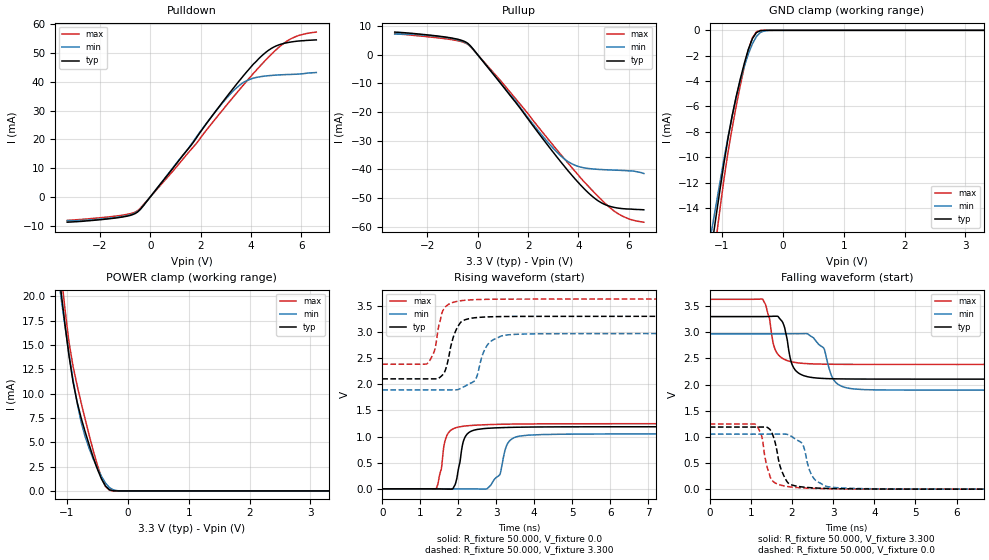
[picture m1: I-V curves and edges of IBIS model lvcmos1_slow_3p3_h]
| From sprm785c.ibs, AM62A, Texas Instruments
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|   slow_3p3_h
[Model]   lvcmos1_slow_3p3_h
Model_type I/O
Polarity   Non-Inverting
Enable   Active-High
Vinl = 0
Vinh = 0.8
Vmeas = 1.65
Vref = 3.3
Cref = 2pF
Rref = 100000
|   typ   min   max
C_comp   3.477pF   3.396pF   3.491pF
[Voltage Range]   3.3   2.97   3.63
[Temperature Range]   27   150   -40
[Pullup Reference]   3.3   2.97   3.63
[Pulldown Reference]   0   0   0
[Power Clamp Reference]   3.3   2.97   3.63
[GND Clamp Reference]   0   0   0
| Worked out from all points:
|   slope of the pulldown table from 0 to 0.495 V, typ, clamps not added: 90.3 ohm
|   slope of the pullup table from 0 to 0.495 V, typ, clamps not added: 91.7 ohm
|   GND clamp passes 1 mA (typ) near -0.53 V on its own axis
|   POWER clamp passes 1 mA (typ) near -0.41 V on its own axis
|   rising waveform, R_fixture 50.000, V_fixture 0.0: 20-80 % time 183ps typ, 292ps min, 182ps max; typ from 0 V to 1.19 V
|   rising waveform, R_fixture 50.000, V_fixture 3.300: 20-80 % time 266ps typ, 306ps min, 208ps max; typ from 2.1 V to 3.3 V
|   falling waveform, R_fixture 50.000, V_fixture 3.300: 20-80 % time 198ps typ, 329ps min, 206ps max; typ from 3.3 V to 2.1 V
|   falling waveform, R_fixture 50.000, V_fixture 0.0: 20-80 % time 245ps typ, 257ps min, 194ps max; typ from 1.19 V to 0 V
[Pulldown]
|Voltage   I(typ)   I(min)   I(max)
-3.3V     -8.786mA   -8.326mA   -8.158mA
-1.3V     -7.238mA   -7.068mA   -6.584mA
-500mV    -5.218mA   -5.082mA   -4.783mA
-300mV    -3.329mA   -3.373mA   -2.999mA
1.6V      17.7mA     17.93mA    16.27mA
2.7V      30.97mA    30.86mA    28.33mA
3.2V      36.66mA    35.95mA    33.67mA
3.6V      41.04mA    39.17mA    37.86mA
4.3V      47.96mA    41.7mA     44.88mA
4.9V      52.07mA    42.31mA    50.35mA
5.7V      54.01mA    42.64mA    55.45mA
6.6V      54.61mA    43.26mA    57.33mA
[Pullup]
|Voltage   I(typ)   I(min)   I(max)
-3.3V     7.94mA     7.245mA    7.375mA
-1.4V     6.356mA    6.223mA    5.749mA
-800mV    5.458mA    5.239mA    4.924mA
-400mV    4.045mA    3.827mA    3.712mA
1V        -10.95mA   -10.84mA   -9.98mA
2.7V      -30.6mA    -29.63mA   -28.35mA
3.5V      -39.5mA    -36.72mA   -36.87mA
4.1V      -45.55mA   -39.2mA    -43.06mA
4.9V      -51.56mA   -40.02mA   -50.44mA
5.4V      -53.19mA   -40.22mA   -54.38mA
5.7V      -53.63mA   -40.32mA   -56.03mA
6.6V      -54.06mA   -41.4mA    -58.4mA
[GND_clamp]
|Voltage   I(typ)   I(min)   I(max)
-3.3V     -113.8mA   -82.24mA   -159mA
-1.167V   -17.01mA   -15.72mA   -19.19mA
-1.1V     -14.77mA   -13.85mA   -16.62mA
-1.033V   -12.58mA   -11.98mA   -14.1mA
-900mV    -8.5mA     -8.403mA   -9.586mA
-767mV    -5.246mA   -5.262mA   -5.996mA
-700mV    -3.866mA   -3.96mA    -4.363mA
-567mV    -1.506mA   -1.869mA   -1.555mA
-500mV    -657.8uA   -1.066mA   -589.2uA
-433mV    -173.4uA   -482uA     -106.1uA
-233mV    -388.4nA   -7.967uA   -203.5nA
3.3V      0A         0A         0A
[POWER_clamp]
|Voltage   I(typ)   I(min)   I(max)
-3.3V     168.5mA    143.2mA    197.8mA
-1.1V     20.63mA    20.01mA    22.62mA
-1.033V   17.13mA    16.96mA    18.7mA
-967mV    13.91mA    14.09mA    15.3mA
-900mV    11.2mA     11.42mA    12.8mA
-767mV    7.499mA    7.079mA    9.068mA
-633mV    4.696mA    4.33mA     5.685mA
-500mV    2.241mA    2.319mA    2.654mA
-367mV    495uA      804.4uA    468.5uA
-300mV    111.9uA    329.7uA    65.22uA
-100mV    170.1nA    4.018uA    96.08nA
3.3V      0A         0A         0A
[Ramp]
| variable   typ   min   max
dV/dt_r   0.713/0.182n   0.631/0.292n   0.747/0.181n
dV/dt_f   0.718/0.197n   0.647/0.329n   0.747/0.207n
R_load = 50.000
[Rising Waveform]
R_fixture= 50.000
V_fixture= 0.0
V_fixture_min= 0.0
V_fixture_max= 0.0
|time   V(typ)   V(min)   V(max)
0s        2.269uV    23.11uV    3.249uV
1.417ns   -521.6uV   104.5uV    1.015mV
1.679ns   -4.773mV   -51.5uV    981.7mV
1.917ns   77.09mV    -332.5uV   1.163V
2.073ns   664mV      -1.539mV   1.19V
2.234ns   1.047V     -1.716mV   1.205V
2.761ns   1.157V     3.043mV    1.228V
3.307ns   1.174V     874.2mV    1.237V
3.607ns   1.179V     1.008V     1.24V
10ns      1.188V     1.052V     1.246V
[Rising Waveform]
R_fixture= 50.000
V_fixture= 3.300
V_fixture_min= 2.970
V_fixture_max= 3.630
|time   V(typ)   V(min)   V(max)
0s        2.103V     1.892V     2.385V
1.184ns   2.103V     1.892V     2.396V
1.376ns   2.103V     1.893V     2.644V
1.497ns   2.121V     1.892V     3.143V
1.644ns   2.24V      1.892V     3.465V
2.012ns   3.129V     1.904V     3.592V
2.445ns   3.273V     2.081V     3.619V
2.79ns    3.289V     2.772V     3.625V
3.21ns    3.296V     2.936V     3.628V
10ns      3.3V       2.97V      3.63V
[Falling Waveform]
R_fixture= 50.000
V_fixture= 3.300
V_fixture_min= 2.970
V_fixture_max= 3.630
|time   V(typ)   V(min)   V(max)
0s        3.3V       2.97V      3.63V
1.289ns   3.3V       2.97V      3.629V
1.66ns    3.302V     2.97V      2.576V
1.805ns   3.126V     2.97V      2.485V
2.077ns   2.278V     2.972V     2.422V
2.524ns   2.131V     2.891V     2.395V
2.774ns   2.116V     2.692V     2.39V
3.029ns   2.11V      2.073V     2.388V
3.411ns   2.107V     1.925V     2.386V
10ns      2.103V     1.892V     2.385V
[Falling Waveform]
R_fixture= 50.000
V_fixture= 0.0
V_fixture_min= 0.0
V_fixture_max= 0.0
|time   V(typ)   V(min)   V(max)
0s        1.188V     1.052V     1.246V
1.106ns   1.188V     1.052V     1.241V
1.265ns   1.188V     1.052V     1.011V
1.418ns   1.171V     1.052V     364.5mV
1.547ns   1.002V     1.052V     143.1mV
1.873ns   150.2mV    1.05V      52.67mV
2.237ns   43.23mV    881.6mV    24.44mV
2.474ns   26.95mV    277.4mV    16.29mV
2.851ns   14.17mV    50.22mV    9.394mV
10ns      63.6uV     132.8uV    38.55uV
